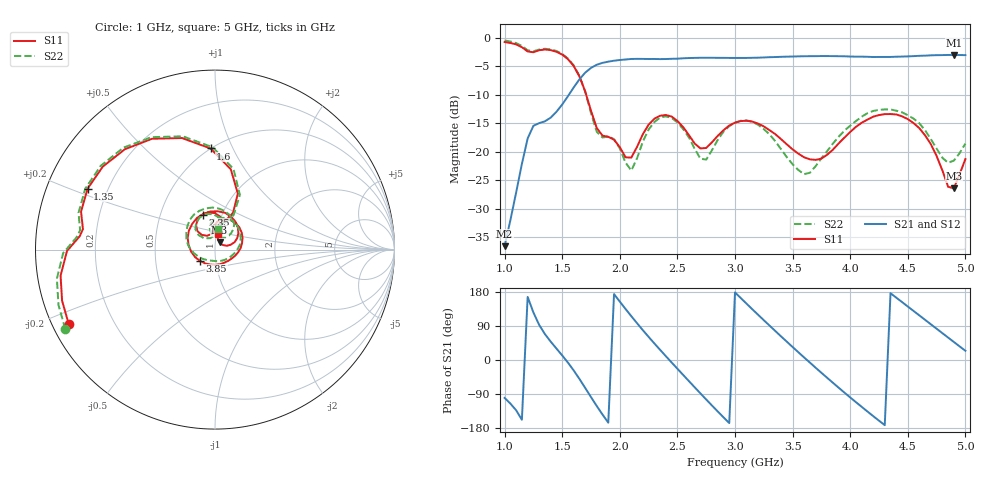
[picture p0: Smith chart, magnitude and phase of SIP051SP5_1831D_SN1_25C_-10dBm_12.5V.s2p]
# GHz  S  dB  R  50
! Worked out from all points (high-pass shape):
!   81 points, 1 GHz to 5 GHz, reference 50 ohm
!   highest |S21| = -3.03 dB at 4.9 GHz (marker M1); lowest = -36.5 dB at 1 GHz (marker M2)
!   |S21| within 3 dB of the highest: 1.706 GHz to end of sweep
!   lowest |S11| = -26.4 dB at 4.9 GHz (marker M3), VSWR 1.10, Z = 52.4 + j4.27 ohm
!   |S11| at or under -10 dB: 1.708 GHz to end of sweep
!   |S22| runs from -23.9 to -0.5 dB; largest |S21 - S12| = 0.0023
!   S11 on the Smith chart (normalised r, x): 1 GHz: 0.05, -0.24; 1.35 GHz: 0.13, +0.22; 1.6 GHz: 0.50, +0.82; 2.35 GHz: 0.81, +0.33; 3.85 GHz: 0.84, -0.11; 5 GHz: 1.02, +0.17
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1  -0.77 -152.9  -36.53 -100.0  -36.66 -100.7  -0.50 -152.0
1.2  -2.42 174.3  -17.66 166.5  -17.66 166.4  -2.21 175.0
1.35  -2.08 154.4  -14.66 68.4  -14.63 68.4  -1.95 154.8
1.6  -4.97 92.5  -8.72 -27.6  -8.72 -27.6  -4.87 91.4
1.7  -9.45 67.8  -6.13 -73.8  -6.14 -73.8  -9.51 65.6
1.8  -15.84 71.6  -4.75 -121.5  -4.76 -121.5  -16.50 71.1
1.95  -17.89 90.7  -4.04 173.9  -4.05 174.0  -17.78 89.2
2.15  -19.13 132.1  -3.72 97.0  -3.72 97.0  -21.12 134.1
2.35  -13.68 109.7  -3.76 26.8  -3.75 26.8  -14.01 114.6
2.5  -14.59 81.4  -3.69 -23.0  -3.68 -23.0  -14.85 83.1
2.7  -19.41 79.3  -3.53 -88.2  -3.53 -88.1  -21.21 79.4
3  -14.89 71.1  -3.56 178.4  -3.55 178.6  -14.93 81.4
3.2  -15.06 32.6  -3.51 119.5  -3.51 119.5  -15.27 36.5
3.35  -16.91 3.1  -3.40 76.5  -3.40 76.6  -18.16 -0.9
3.55  -20.32 -40.9  -3.28 20.5  -3.28 20.5  -23.19 -67.2
3.7  -21.41 -87.8  -3.25 -20.4  -3.24 -20.3  -22.52 -130.1
3.85  -19.63 -142.9  -3.24 -60.1  -3.23 -60.2  -18.57 -169.8
4.05  -15.62 156.9  -3.33 -111.3  -3.32 -111.2  -14.61 149.4
4.35  -13.39 85.7  -3.38 176.2  -3.38 176.3  -12.59 92.9
4.65  -17.11 27.3  -3.15 106.0  -3.15 106.1  -16.23 48.3
4.9  -26.40 58.0  -3.03 47.5  -3.03 47.5  -21.54 72.7
5  -21.28 78.2  -3.07 24.3  -3.08 24.4  -18.56 80.6
